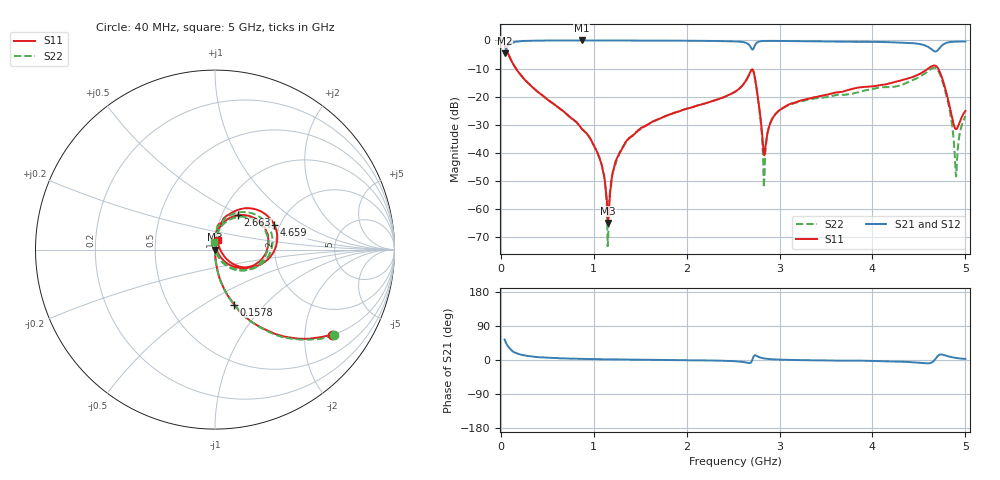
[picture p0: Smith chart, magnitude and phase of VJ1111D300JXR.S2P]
! VJ1111D300JXR
! DATE 02/16/2022  10:22
! CAPACITORS MOUNTED IN SERIES ON 25 MIL THICK MICROSTRIP SUBSTRATE
# GHz  S  MA  R  50.00
!  FREQ  S11M  S11A  S21M  S21A  S12M  S12A  S22M  S22A
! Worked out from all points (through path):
!   801 points, 40 MHz to 5 GHz, reference 50 ohm
!   highest |S21| = -0.01 dB at 870.8 MHz (marker M1); lowest = -4.6 dB at 40 MHz (marker M2)
!   group delay of S21, straight-line fit = 6.28 ps
!   lowest |S11| = -64.9 dB at 1.156 GHz (marker M3), VSWR 1.00, Z = 50.1 + j0.012 ohm
!   |S11| at or under -10 dB: 162 MHz to 4.599 GHz (4.437 GHz wide, 186 % of centre); 4.707 GHz to end of sweep
!   |S22| runs from -73.1 to -1.8 dB; largest |S21 - S12| = 0.037
!   S11 on the Smith chart (normalised r, x): 40 MHz: 1.01, -2.74; 157.8 MHz: 1.00, -0.69; 2.663 GHz: 1.19, +0.48; 4.659 GHz: 1.86, +0.59; 5 GHz: 1.03, +0.11
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0.04  0.8068 -36.0  0.5869 54.0  0.5876 54.2  0.8158 -35.7
0.1578  0.3239 -70.8  0.9448 19.1  0.9451 20.0  0.3261 -70.8
0.8708  0.02696 -87.6  0.9985 2.9  1.003 2.7  0.02682 -88.1
1.0692  0.007404 -87.4  0.997 2.1  1.003 1.9  0.007424 -91.0
1.1126  0.003815 -82.7  0.9968 1.9  1.003 1.7  0.003605 -96.8
1.1374  0.00172 -77.3  0.9964 1.9  1.001 1.7  0.001358 -84.9
1.156  0.0005712 12.1  0.9968 1.8  1.002 1.6  0.0003077 96.9
1.2056  0.004638 86.2  0.9959 1.6  1.002 1.4  0.004631 85.0
1.2986  0.01147 87.3  0.996 1.4  1.002 1.1  0.012 88.1
1.6954  0.03987 87.7  0.9916 0.4  0.9975 0.1  0.0399 86.6
2.52  0.1223 78.5  0.9611 -3.2  0.9675 -3.5  0.1219 76.8
2.6626  0.2296 56.3  0.8606 -7.9  0.8658 -8.0  0.2287 53.1
2.7308  0.2337 -22.1  0.7912 12.2  0.7959 12.0  0.2297 -27.7
2.8362  0.009121 22.6  0.9789 4.0  0.9849 3.9  0.003709 69.9
2.8858  0.02905 82.1  0.9813 2.6  0.9875 2.4  0.02885 94.7
2.954  0.04905 87.0  0.98 1.5  0.9862 1.3  0.04869 91.5
3.3508  0.09578 85.2  0.9662 -0.8  0.9718 -0.9  0.09138 85.5
4.1754  0.1707 75.2  0.9319 -3.7  0.938 -3.9  0.1475 74.3
4.659  0.3578 22.6  0.6514 -2.7  0.6549 -2.7  0.3271 20.3
4.7954  0.1174 -39.2  0.9052 11.1  0.9102 11.0  0.1055 -53.1
4.8946  0.02668 14.0  0.9537 5.6  0.9587 5.5  0.004465 -16.7
5  0.05601 73.2  0.9574 2.8  0.9636 2.7  0.0449 93.9
